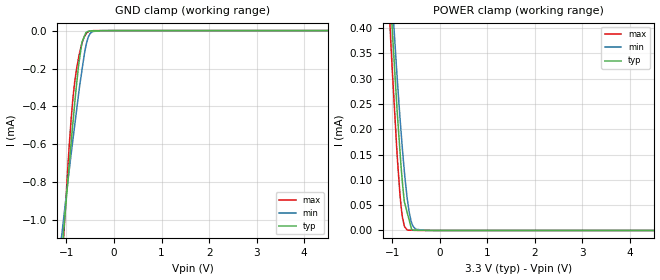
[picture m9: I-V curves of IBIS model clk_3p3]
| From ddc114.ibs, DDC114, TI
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|   clk_3p3 Model
[Model]   clk_3p3
Model_type   Input
Vinl = 0.66
Vinh = 2.64
|   typ   min   max
|   (nom PVT)   (fast PVT)   (slow PVT)
|C_comp from frequency sweep method (F=19.2MHz)
|Average
|C_comp   5.438e-13   4.672e-13   6.230e-13
|C_comp from LC tank measurement(L=1nH)
|Average
|Resonant Frequency(Hz)   5.241e+10   6.068e+10   3.033e+10
C_comp   9.231e-15   6.886e-15   2.756e-14
| Where nom  PVT is Nominal Process, 3.3V, 27C
|   Fast PVT is Strong Process,  3.6V, -40C
|   Slow PVT is Weak Process,   3V, 87C
[Model Spec]
|Subparameter   typ   min   max
Vinl   0.66   0.60   0.72
Vinh   2.64   2.4   2.88
[Voltage Range]   3.3   3   3.6
|Ambient Temperature   25   85   -40
|Junction Temperature
[Temperature Range]   27   87   -40
[Power Clamp Reference]   3.3   3   3.6
[GND Clamp Reference]   0   0   0
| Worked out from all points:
|   GND clamp passes 1 mA (typ) near -1.04 V on its own axis
|   POWER clamp passes 1 mA (typ) near -1.34 V on its own axis
[GND Clamp]
|   Voltage   I(typ)   I(min)   I(max)
-3.3V     -8.269mA   -6.097mA   -11.78mA
-1.087V   -1.148mA   -1.054mA   -1.214mA
-1.02V    -940.7uA   -906.9uA   -929.1uA
-972mV    -800.4uA   -802.7uA   -728.4uA
-896.4mV  -578.2uA   -642.2uA   -453.9uA
-824.4mV  -380.7uA   -497.1uA   -268.1uA
-745.8mV  -186.9uA   -338.7uA   -146.8uA
-673.2mV  -61.7uA    -209.5uA   -66.34uA
-554.4mV  -5.364uA   -46.05uA   -8.12uA
-456mV    -2.01uA    -5.772uA   -813.1nA
-285mV    -1.25uA    -60.06nA   -147.6nA
6.6V      0A         0A         0A
[POWER Clamp]
|   Voltage   I(typ)   I(min)   I(max)
-3.3V     4.912mA    4.599mA    5.321mA
-1.145V   644.9uA    683.9uA    592.5uA
-1.026V   440uA      493.9uA    366.1uA
-1.004V   405.5uA    461.5uA    326.4uA
-897.6mV  237.4uA    303.9uA    150.1uA
-835.2mV  154.2uA    220.6uA    69.04uA
-788.4mV  97.9uA     164uA      27.92uA
-745.8mV  57.01uA    118uA      9.29uA
-684mV    34.98uA    62.53uA    950.2nA
-561mV    709.3nA    8.136uA    368.2nA
-285mV    358.3nA    0A         0A
6.6V      0A         0A         0A
